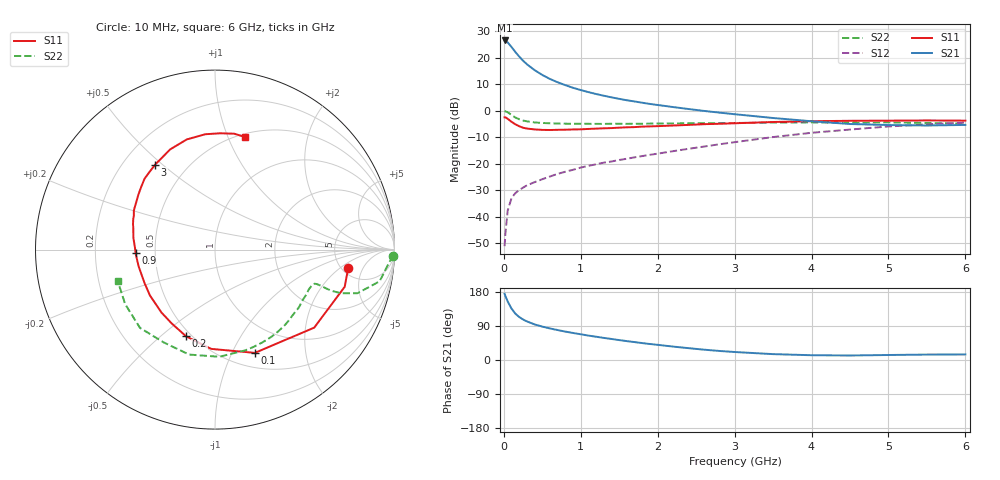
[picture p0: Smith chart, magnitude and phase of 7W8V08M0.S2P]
! Infineon Technologies  Discrete & RF Semiconductors
! BFS17W
! Si NPN RF Bipolar Junction Transistor in SOT323
! VCE = 8 V  IC = 8 mA
! Common Emitter S-Parameters:  August  1999
# GHz  S  MA  R  50
!  f  S11  S21  S12  S22
! GHz  MAG  ANG  MAG  ANG  MAG  ANG  MAG  ANG
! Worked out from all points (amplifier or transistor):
!   36 points, 10 MHz to 6 GHz, reference 50 ohm
!   highest |S21| = 26.5 dB at 10 MHz (marker M1)
!   |S21| within 3 dB of that: start of sweep to 113.9 MHz
!   unconditionally stable (mu >= 1): 474.2 MHz to 2.226 GHz; 5.394 GHz to end of sweep
!   at 250 MHz: K = 0.72, MSG = 23.9 dB, |S12| = -29.0 dB
!   at 1.4 GHz: K = 1.18, MAG = 9.5 dB, |S12| = -19.1 dB
!   at 6 GHz: K = 1.04, MAG = -1.7 dB, |S12| = -4.5 dB
!   S11 on the Smith chart (normalised r, x): 10 MHz: 5.71, -2.65; 100 MHz: 0.66, -1.23; 200 MHz: 0.47, -0.61; 900 MHz: 0.39, -0.02; 3 GHz: 0.33, +0.47; 6 GHz: 0.53, +1.15
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0.01  0.7492 -7.8  21.05 174.8  0.0028 82.3  0.993 -1.9
0.02  0.7518 -16.0  20.93 169.1  0.0048 85.3  0.9696 -4.7
0.05  0.7032 -38.2  19.32 154.4  0.0131 74.4  0.934 -10.9
0.1  0.6167 -68.9  15.83 135.5  0.0226 62.1  0.8308 -17.0
0.15  0.5536 -92.2  12.74 122.2  0.028 56.2  0.7436 -19.1
0.2  0.5094 -108.4  10.47 113.4  0.032 55.3  0.6886 -19.5
0.25  0.4767 -120.5  8.744 106.9  0.0355 53.2  0.6511 -19.2
0.3  0.4603 -130.4  7.494 101.8  0.0392 55.0  0.6296 -18.9
0.4  0.4435 -144.8  5.797 93.9  0.045 56.4  0.6005 -18.7
0.5  0.4347 -154.5  4.711 88.1  0.0512 59.0  0.5871 -18.9
0.6  0.4324 -161.8  3.954 83.2  0.0576 60.8  0.5785 -19.6
0.7  0.4358 -167.8  3.429 79.0  0.0645 62.9  0.5737 -20.8
0.9  0.4428 -177.3  2.697 71.3  0.077 65.3  0.5669 -23.7
1.1  0.4529 174.7  2.237 64.4  0.0914 66.4  0.566 -27.2
1.3  0.4655 167.9  1.913 58.3  0.1049 67.5  0.5641 -31.3
1.6  0.4863 159.5  1.571 49.8  0.1244 69.3  0.5656 -37.6
2.2  0.5252 144.4  1.171 35.4  0.1726 71.9  0.5759 -52.2
3  0.5791 125.1  0.858 21.1  0.2552 70.8  0.5861 -73.2
3.5  0.6117 114.1  0.728 15.5  0.3185 67.5  0.5975 -87.7
4.5  0.6449 94.8  0.561 11.9  0.441 55.8  0.5909 -119.1
5.5  0.6546 80.6  0.526 14.3  0.5524 42.6  0.5856 -148.7
6  0.649 75.1  0.539 14.7  0.5962 36.0  0.5696 -162.1
